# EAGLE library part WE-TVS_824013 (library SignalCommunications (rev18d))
TVS Diode High Speed Series Characteristics Low clamping voltage Sturdy design Very low capacitance Flow Thru Design for a simple layout Rail to Rail protection Epoxy flame resistant UL94 V-0 RoHS, REACH and free of halogens Applications Very fast data lines USB 2.0 Ethernet PoE VGA Sim Cards Keypads ESD protection in accordance with EN 61000-4-2, – 8 kV contact discharge – 15 kV air discharge Details see: http://katalog.we-online.de/en/pbs/WE-TVS_High_Speed/824001? Updated by Dan Xu 2014-07-11 2014 (C) Wurth Elektronik
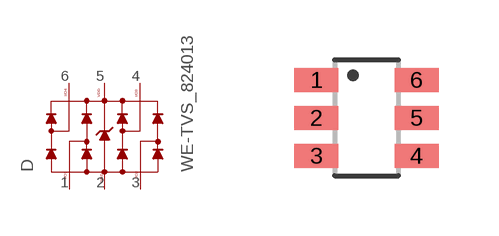
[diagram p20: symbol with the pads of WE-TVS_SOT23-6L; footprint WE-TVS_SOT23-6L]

Designator prefix D

## WE-TVS_824013  [WE-TVS_SOT23-6L]
1  1
2  GND  pwr
3  3
4  4
5  VDD  pwr
6  6

## Footprint WE-TVS_SOT23-6L (pad centres in mm)
TVS Diode Array WE-TVS
smd 1.1 x 0.6: 1 -1.25,0.95; 2 -1.25,0; 3 -1.25,-0.95; 4 1.25,-0.95; 5 1.25,0; 6 1.25,0.95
